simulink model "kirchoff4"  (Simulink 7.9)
settings: Solver=ode23s  StartTime=0.0  StopTime=1  RelTol=1e-3
libraries: fl_lib x14, nesl_utility x8, powerlib x1

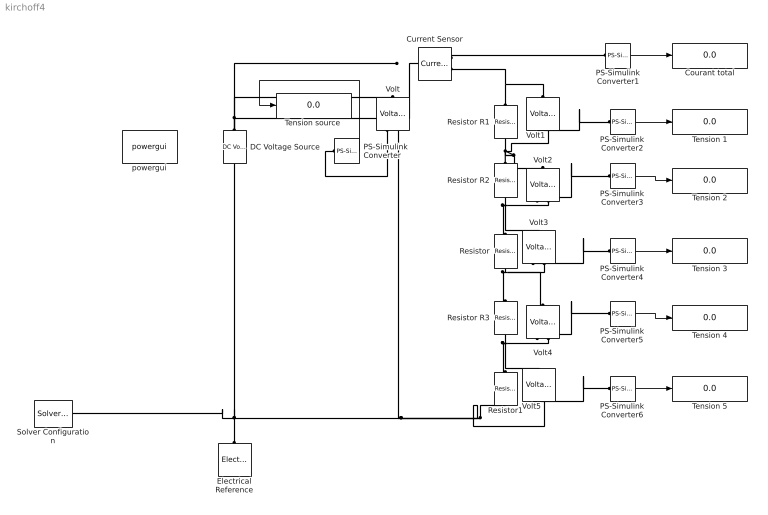
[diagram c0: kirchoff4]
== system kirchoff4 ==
  Courant total : Display
  Current Sensor : fl_lib/Electrical/Electrical Sensors/Current Sensor  i1_Log=off  v1_Log=off  LocalVarNames=|i1|v1  LocalVarDescs=|i1|v1  LocalVarLogging=[0 0]
  DC Voltage Source : fl_lib/Electrical/Electrical Sources/DC Voltage Source  v0=10 V  i_Log=off  v_Log=off  LocalVarNames=|i|v  LocalVarDescs=|i|v  LocalVarLogging=[0 0]
  Electrical Reference : fl_lib/Electrical/Electrical Elements/Electrical Reference  i_Log=off  LocalVarNames=|i  LocalVarDescs=|i  LocalVarLogging=0
  PS-Simulink Converter{,2..6} (6 alike) : nesl_utility/PS-Simulink Converter  PhysicalDomain=network_engine_domain  LeftPortType=input  RightPortType=output  SubClassName=ps_output  Unit=V  AffineConversion=off
  PS-Simulink Converter1 : nesl_utility/PS-Simulink Converter  PhysicalDomain=network_engine_domain  LeftPortType=input  RightPortType=output  SubClassName=ps_output  Unit=A  AffineConversion=off
  Resistor : fl_lib/Electrical/Electrical Elements/Resistor  R=100 Ohm  i_Log=off  v_Log=off  LocalVarNames=|i|v  LocalVarDescs=|i|v  LocalVarLogging=[0 0]
  Resistor R1 : fl_lib/Electrical/Electrical Elements/Resistor  R=100 Ohm  i_Log=off  v_Log=off  LocalVarNames=|i|v  LocalVarDescs=|i|v  LocalVarLogging=[0 0]
  Resistor R2 : fl_lib/Electrical/Electrical Elements/Resistor  R=100 Ohm  i_Log=off  v_Log=off  LocalVarNames=|i|v  LocalVarDescs=|i|v  LocalVarLogging=[0 0]
  Resistor R3 : fl_lib/Electrical/Electrical Elements/Resistor  R=100 Ohm  i_Log=off  v_Log=off  LocalVarNames=|i|v  LocalVarDescs=|i|v  LocalVarLogging=[0 0]
  Resistor1 : fl_lib/Electrical/Electrical Elements/Resistor  R=100 Ohm  i_Log=off  v_Log=off  LocalVarNames=|i|v  LocalVarDescs=|i|v  LocalVarLogging=[0 0]
  Solver Configuration : nesl_utility/Solver Configuration  PhysicalDomain=network_engine_domain  LeftPortType=input  RightPortType=generic  SubClassName=solver  UseCustomDae=off  DoDC=off  ResidualTolerance=1e-9  UseLocalSolver=off  LocalSolverChoice=NE_BACKWARD_EULER_ADVANCER  LocalSolverSampleTime=.001  DoFixedCost=off  MaxNonlinIter=3  MaxModeIter=2  LinearAlgebra=Sparse  Accelerate=off  Profile=off  UseLocalSampling=off  DelaysMemoryBudget=1024
  Tension {1..5} (5 alike) : Display
  "Tension source " : Display
  Volt{,1..5} (6 alike) : fl_lib/Electrical/Electrical Sensors/Voltage Sensor  i1_Log=off  v1_Log=off  LocalVarNames=|i1|v1  LocalVarDescs=|i1|v1  LocalVarLogging=[0 0]
  powergui : powerlib/powergui  Priority=1  SimulationMode=Continuous  SolverType=Tustin  SampleTime=50e-6  frequency=60  SPID=off  DisableSnubberDevices=off  DisableRonSwitches=off  DisableVfSwitches=off  SwTol=0  Interpol=off  DisplayEquations=off  FunctionMessages=off  frequencyindice=17  Pbase=100e6  ErrMax=1e-4  Iterations=50  UnitsV=V  UnitsW=W  echomessages=off  HookPort=off  EnableUseOfTLC=off  x0status=blocks  RestoreLinks=warning  ResistiveCurrentMeasurement=off  Ylog=off  Xlog=on  ShowGrid=off  save=off  variable=ZData  ZoomFFT=off  StartTime=0.0  cycles=1  DisplayStyle=1  FreqAxis=off  MaxFrequency=1000  frequencyindicesteady=1  display=off  methode=off
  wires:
  PS-Simulink Converter1/1 -> Courant total/1
  PS-Simulink Converter/1 -> "Tension source "/1
  PS-Simulink Converter2/1 -> Tension 1/1
  PS-Simulink Converter3/1 -> Tension 2/1
  PS-Simulink Converter4/1 -> Tension 3/1
  PS-Simulink Converter5/1 -> Tension 4/1
  PS-Simulink Converter6/1 -> Tension 5/1
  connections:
  DC Voltage Source/LConn1 -- Volt/LConn1 -- Current Sensor/LConn1
  Current Sensor/RConn1 -- PS-Simulink Converter1/LConn1
  Resistor R1/LConn1 -- Current Sensor/RConn2 -- Volt1/LConn1
  Volt/RConn1 -- PS-Simulink Converter/LConn1
  Volt1/RConn1 -- PS-Simulink Converter2/LConn1
  Volt3/RConn1 -- PS-Simulink Converter4/LConn1
  Volt2/RConn1 -- PS-Simulink Converter3/LConn1
  Resistor R2/LConn1 -- Volt1/RConn2 -- Resistor R1/RConn1 -- Volt2/LConn1
  Volt2/RConn2 -- Volt3/LConn1 -- Resistor R2/RConn1 -- Resistor/LConn1
  Volt4/RConn2 -- Resistor1/LConn1 -- Resistor R3/RConn1 -- Volt5/LConn1
  Volt4/RConn1 -- PS-Simulink Converter5/LConn1
  Volt5/RConn1 -- PS-Simulink Converter6/LConn1
  Resistor1/RConn1 -- Volt5/RConn2 -- Electrical Reference/LConn1 -- DC Voltage Source/RConn1 -- Solver Configuration/RConn1 -- Volt/RConn2
  Volt3/RConn2 -- Resistor/RConn1 -- Resistor R3/LConn1 -- Volt4/LConn1
